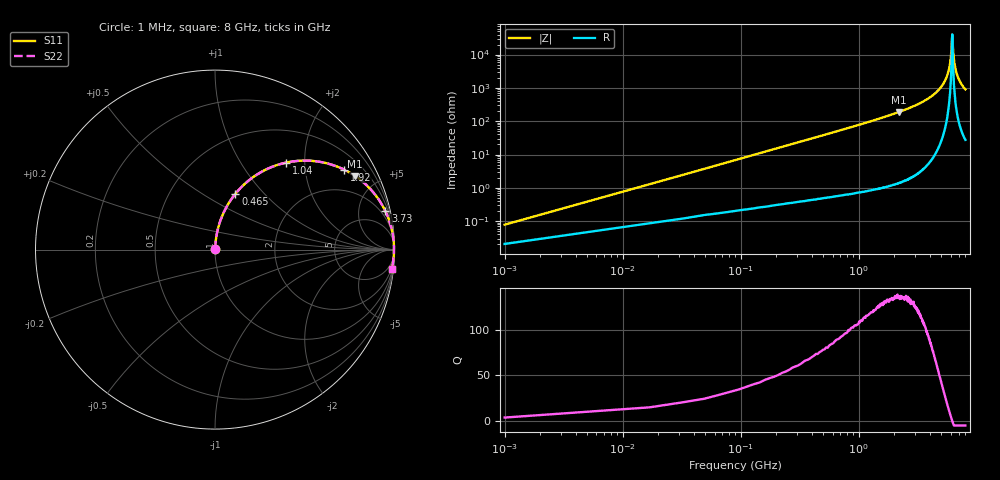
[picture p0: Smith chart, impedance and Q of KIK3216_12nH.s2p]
!version-2
!date-01.2022
!Series
# MHz S RI R 50
!Freq ReS11 ImS11 ReS21 ImS21 ReS12 ImS12 ReS22 ImS22
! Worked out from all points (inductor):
!   501 points, 1 MHz to 8 GHz, reference 50 ohm
!   read as one part in series: L = 12 nH near 33 MHz
!   highest Q = 136 at 2.19 GHz (marker M1), where L = 13.7 nH
!   self-resonance near 6.18 GHz
!   S11 on the Smith chart (normalised r, x): 1 MHz: 1.00, +0.00; 465 MHz: 1.01, +0.71; 1.04 GHz: 1.01, +1.62; 1.92 GHz: 1.02, +3.21; 3.73 GHz: 1.09, +8.83; 8 GHz: 2, -18
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1  0.000215 0.000754  0.9998 -0.000754  0.9998 -0.000754  0.000215 0.000754
49  0.00286 0.0368  0.9971 -0.0368  0.9971 -0.0368  0.00286 0.0368
97  0.0074 0.0725  0.9926 -0.0725  0.9926 -0.0725  0.0074 0.0725
241  0.0351 0.175  0.9649 -0.175  0.9649 -0.175  0.0351 0.175
465  0.1138 0.311  0.8862 -0.311  0.8862 -0.311  0.1138 0.311
1040  0.3958 0.4845  0.6042 -0.4845  0.6042 -0.4845  0.3958 0.4845
1340  0.5309 0.4949  0.4691 -0.4949  0.4691 -0.4949  0.5309 0.4949
1920  0.7183 0.4461  0.2817 -0.4461  0.2817 -0.4461  0.7183 0.4461
2190  0.7797 0.4108  0.2203 -0.4108  0.2203 -0.4108  0.7797 0.4108
2670  0.858 0.3453  0.142 -0.3453  0.142 -0.3453  0.858 0.3453
3730  0.9492 0.2146  0.0508 -0.2146  0.0508 -0.2146  0.9492 0.2146
4020  0.9628 0.1836  0.0372 -0.1836  0.0372 -0.1836  0.9628 0.1836
5350  0.9938 0.0626  0.00619 -0.0626  0.00619 -0.0626  0.9938 0.0626
5700  0.9964 0.0355  0.00359 -0.0355  0.00359 -0.0355  0.9964 0.0355
5940  0.9973 0.0179  0.00272 -0.0179  0.00272 -0.0179  0.9973 0.0179
6050  0.9975 0.00989  0.00253 -0.00989  0.00253 -0.00989  0.9975 0.00989
6190  0.9975 -0.000138  0.00248 0.000138  0.00248 0.000138  0.9975 -0.000138
6230  0.9975 -0.00233  0.0025 0.00233  0.0025 0.00233  0.9975 -0.00233
6350  0.9973 -0.011  0.00267 0.011  0.00267 0.011  0.9973 -0.011
6670  0.9963 -0.0319  0.0037 0.0319  0.0037 0.0319  0.9963 -0.0319
7230  0.9926 -0.0662  0.00736 0.0662  0.00736 0.0662  0.9926 -0.0662
8000  0.9846 -0.1089  0.0154 0.1089  0.0154 0.1089  0.9846 -0.1089
